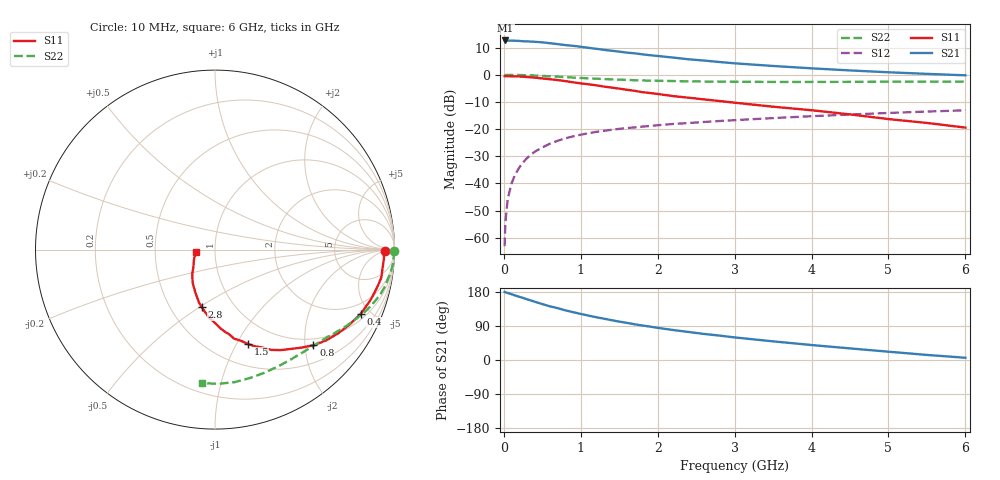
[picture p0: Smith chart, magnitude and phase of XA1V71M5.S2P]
! SIEMENS Discrete & RF Semiconductors
! BFY180
! Si NPN RF Bipolar Junction Transistor in MICRO-X
! VCE = 1.75 V  IC = 1.5 mA
! Common Emitter S-Parameters:  May  1997
# GHz  S  MA  R  50
!  f  S11  S21  S12  S22
! GHz  MAG  ANG  MAG  ANG  MAG  ANG  MAG  ANG
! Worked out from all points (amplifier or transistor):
!   36 points, 10 MHz to 6 GHz, reference 50 ohm
!   highest |S21| = 12.6 dB at 20 MHz (marker M1)
!   |S21| within 3 dB of that: start of sweep to 1.181 GHz
!   unconditionally stable (mu >= 1): 2.853 GHz to end of sweep
!   at 250 MHz: K = 0.12, MSG = 22.3 dB, |S12| = -32.3 dB
!   at 1.4 GHz: K = 0.65, MSG = 14.6 dB, |S12| = -20.3 dB
!   at 6 GHz: K = 1.09, MAG = 4.6 dB, |S12| = -13.1 dB
!   S11 on the Smith chart (normalised r, x): 10 MHz: 34, -5; 400 MHz: 1.30, -4.38; 800 MHz: 0.85, -2.18; 1.5 GHz: 0.73, -1.11; 2.8 GHz: 0.71, -0.51; 6 GHz: 0.81, -0.02
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0.01  0.9444 -0.5  4.241 179.5  0.0007 79.8  0.9957 -0.3
0.02  0.9418 -1.0  4.29 178.6  0.0019 91.1  0.9965 -0.6
0.05  0.9424 -3.1  4.25 176.9  0.0051 85.8  0.996 -1.5
0.1  0.9393 -6.3  4.259 173.6  0.01 86.9  0.9956 -3.1
0.15  0.9394 -9.5  4.234 170.2  0.0149 84.5  0.9944 -4.7
0.25  0.92 -15.2  4.146 163.8  0.0243 80.3  0.987 -7.8
0.4  0.8875 -23.8  4.057 153.9  0.0383 74.8  0.9698 -12.1
0.5  0.8573 -29.3  3.963 147.6  0.0461 70.9  0.9555 -14.9
0.6  0.8293 -34.3  3.817 141.5  0.0539 67.7  0.9396 -17.4
0.8  0.7651 -44.2  3.523 131.0  0.0678 62.1  0.9073 -22.1
0.9  0.7281 -48.6  3.419 126.2  0.0735 59.0  0.8904 -24.2
1.1  0.6692 -56.8  3.14 117.2  0.0841 54.6  0.8607 -28.0
1.3  0.6079 -64.0  2.884 109.1  0.0933 51.0  0.8354 -31.5
1.5  0.5568 -70.8  2.674 101.3  0.1011 48.1  0.8139 -34.7
1.8  0.4793 -80.4  2.383 91.1  0.1113 44.8  0.7884 -39.0
2.2  0.4055 -90.5  2.078 79.1  0.1244 40.6  0.7673 -44.6
2.6  0.3528 -99.0  1.831 68.8  0.1354 37.4  0.7527 -49.8
2.8  0.3297 -102.9  1.723 64.5  0.1409 36.1  0.7474 -52.3
3.5  0.2587 -115.4  1.454 49.2  0.1597 31.2  0.7395 -61.3
4.5  0.1867 -132.8  1.204 30.6  0.1857 23.9  0.7413 -74.5
5.5  0.13 -154.6  1.041 13.4  0.2108 16.1  0.7482 -88.5
6  0.1067 -173.6  0.979 5.9  0.2219 11.9  0.7471 -95.6
